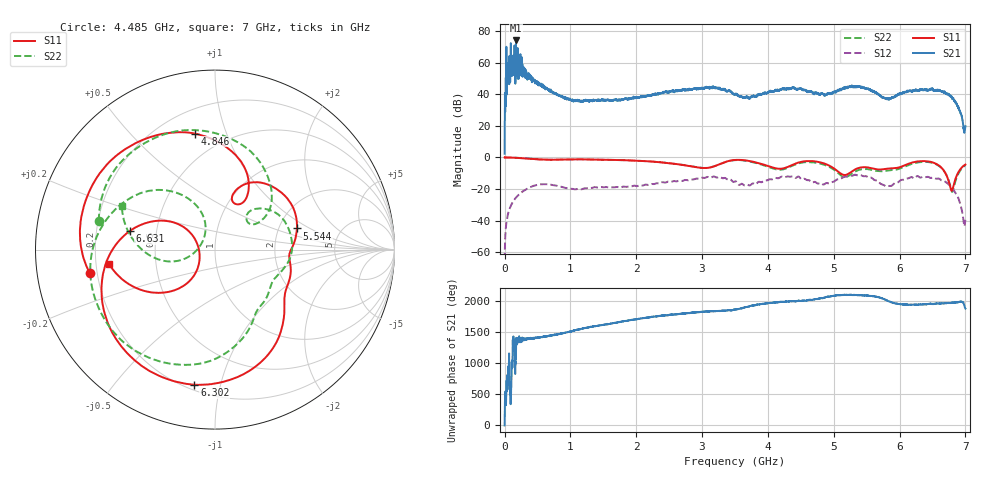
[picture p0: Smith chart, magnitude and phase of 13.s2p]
!Keysight Technologies,N5232A,MY52221221,A.10.65.11
!Date: Wednesday, October 16, 2024 12:04:51
!Correction: S11(Full 2 Port(1,4))
!S41(Full 2 Port(1,4))
!S14(Full 2 Port(1,4))
!S44(Full 2 Port(1,4))
!S2P File: Measurements: S11, S41, S14, S44:
# Hz S  RI  R 50
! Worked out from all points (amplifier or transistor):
!   4001 points, 300 kHz to 7 GHz, reference 50 ohm
!   highest |S21| = 73.9 dB at 173.5 MHz (marker M1)
!   |S21| within 3 dB of that: 94.5698 MHz to 94.93039 MHz (360.6 kHz wide, 0.381 % of centre)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
!   unconditionally stable (mu >= 1): 6.94894 GHz to 6.950947 GHz; 6.951 GHz to end of sweep
!   at 1.166 GHz: K = 2.12, MSG = 27.7 dB, |S12| = -20.1 dB
!   at 3.5 GHz: K = 8.28, MSG = 27.4 dB, |S12| = -15.2 dB
!   at 7 GHz: K = 2.31, MAG = 23.2 dB, |S12| = -39.4 dB
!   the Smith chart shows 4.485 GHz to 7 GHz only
!   S11 on the Smith chart (normalised r, x): 4.485 GHz: 0.17, -0.09; 4.846 GHz: 0.34, +0.78; 5.544 GHz: 2.51, +0.76; 6.302 GHz: 0.23, -0.83; 6.631 GHz: 0.35, +0.09; 7 GHz: 0.25, -0.06
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300000  -0.9957 -0.00956  1.308 -0.1905  -6.09e-05 0.000113  -0.9931 -0.015
6.32973e7  -0.9722 0.2059  -976.9 377.9  0.00547 0.0191  -0.972 0.2119
1.122952e8  -0.9228 0.358  -311.8 -850.3  0.0167 0.0311  -0.9185 0.3668
1.297944e8  -0.8973 0.4055  412.2 -761  0.0218 0.0342  -0.8916 0.4184
1.350442e8  -0.8903 0.4203  943.3 -942.4  0.0234 0.0351  -0.8846 0.4329
1.385441e8  -0.8846 0.43  -467.8 -772.4  0.0246 0.0356  -0.8793 0.4424
1.735426e8  -0.8261 0.5234  -2622 4231  0.0371 0.0393  -0.8179 0.5385
1.85792e8  -0.8022 0.5539  -142.4 -1069  0.042 0.0398  -0.7922 0.57
2.155408e8  -0.7403 0.6222  177 -253.7  0.0539 0.0391  -0.7273 0.6385
3.27536e8  -0.4673 0.8124  174.8 -302.2  0.0984 0.0126  -0.4419 0.8264
5.37527e8  0.0664 0.8618  179.8 -106.4  0.0897 -0.1085  0.1083 0.8589
1.1675e9  0.847 -0.2136  -19.53 55.21  -0.0937 -0.0308  0.8235 -0.2896
2.3347e9  -0.6422 0.3096  68.86 -73.32  0.1343 0.0701  -0.5708 0.4338
3.50015e9  0.7988 -0.235  43.69 85.32  -0.1695 0.0419  0.6971 -0.439
4.485358e9  -0.6976 -0.1321  -145.7 -50.87  0.2305 0.00407  -0.6476 0.1596
4.66735e9  -0.6255 0.4467  -99.24 -64.3  0.1435 -0.0769  -0.3379 0.6207
4.845842e9  -0.1116 0.6465  -39.54 -90.16  0.1009 -0.0959  0.1652 0.5735
5.544062e9  0.4567 0.1181  20.51 -142  -0.1864 0.1342  0.4151 -0.054
5.83455e9  0.4184 -0.1508  -66.75 -16.25  0.1023 -0.073  0.2898 -0.2626
6.30178e9  -0.1143 -0.7532  -109.2 87.03  -0.1001 0.2143  -0.3985 -0.5882
6.630766e9  -0.4762 0.1025  -115.6 48.44  0.1816 0.0617  -0.3472 0.3306
7e9  -0.5915 -0.0782  2.559 9.408  -0.00872 0.00619  -0.5192 0.2434
